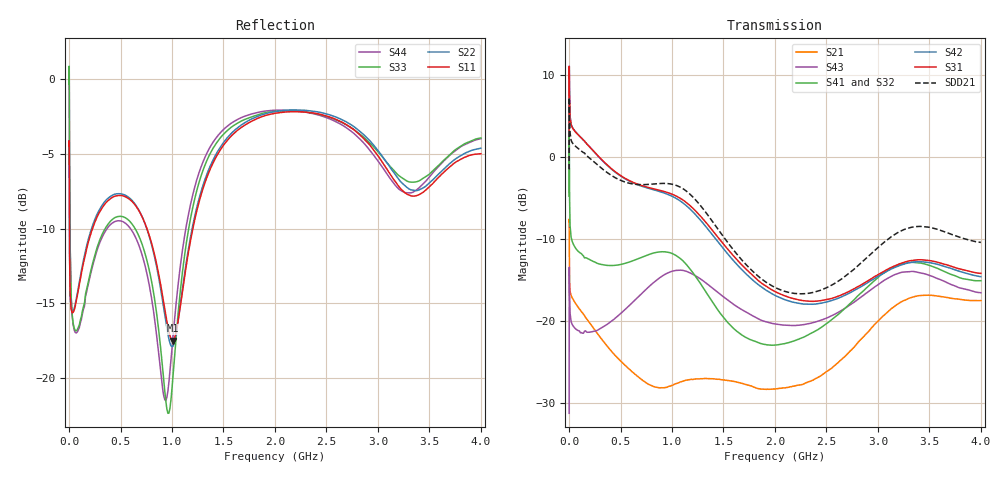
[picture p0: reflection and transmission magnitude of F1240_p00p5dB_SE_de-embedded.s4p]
! Integrated Device Technology
! Corporate Headquarters
! 6024 Silver Creek Valley Road
! San Jose, CA 95138  USA
! Phone:  1-408-284-8200
! Toll Free:  1-800-223-1366
! Webpage:  http://www.idt.com/
! Timing and RF Division
! 515 Groton Road, Suite 102
! Westford, MA 01886-6024
! Device:  F1240
! Description: Dual Intermediate Frequency Digital Variable Gain Amplifier
! Frequency:  10.0 -  500.00 MHz
! Package:  5x5 mm QFN Plastic Package: 32 pin
! Ports:  8 RF, 20 DC
!  Pin  1  = GA3 / Data  Pin 17  = RF OUT_B+
!  Pin  2  = GA4 / CLK  Pin 18  = RF OUT_B-
!  Pin  3  = GA5  Pin 19  = STBY_B
!  Pin  4  = VMODE  Pin 20  = Ground
!  Pin  5  = No Connect  Pin 21  = Ground
!  Pin  6  = GB5  Pin 22  = STB_A
!  Pin  7  = GB4  Pin 23  = RF OUT_A-  = Port 4
!  Pin  8  = GB3  Pin 24  = RF OUT_A+  = Port 3
!  Pin  9  = GB2  Pin 25  = GA0
!  Pin 10  = GB1  Pin 26  = ISET_A
!  Pin 11  = RF IN_B+  Pin 27  = VCC
!  Pin 12  = RF IN_B-  Pin 28  = Ground
!  Pin 13  = Ground  Pin 29  = RF IN_A-  = Port 2
!  Pin 14  = VCC  Pin 30  = RF IN_A+  = Port 1
!  Pin 15  = ISET_B  Pin 31  = GA1
!  Pin 16  = GB0  Pin 32  = GA2 / CSb
! Gain  = +19.5 dB
! State  = 1
! Voltage  = +5.00 V
! Current  = 85.292 mA (one channel only)
! Temperture  =  +25 C
! Test Date  =  2017-10-18
! Board  =  EB4031
! Data:  The device was measured on a custom evaluation board which has
!  individual transmission lines to the RF pins.  Data was collected
!  using a calibrated network analyzer.  The evaluation board was
!  de-embedded using Automatic Fixture Removal.
!  The reference plane is the edge of the package pin.
!  Only Channel A was measured.
!  This data is in single-ended operation.  If your needs are balanced
!  or differential S-parameters then this file needs to be used a
!  linear simulator.
! File Date:  2017-11-10  MJV
! Note:
!  Integrated Device Technology supplies this data as a sample of measured
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# Hz S dB R 100
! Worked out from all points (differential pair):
!   410 points, 500 kHz to 4 GHz, reference 100 ohm
!   strongest paths, dB at 500 kHz, 930 MHz, 1.96 GHz, 2.98 GHz, 4 GHz:
!     S31: 3.0, -4.2, -16.1, -14.5, -14.2
!     S42: 3.0, -4.4, -16.6, -14.7, -14.6
!     S41: -4.8, -11.6, -23.0, -14.9, -15.1
!     S32: -4.8, -11.8, -22.9, -15.3, -15.6
!     S43: -31.3, -14.3, -20.3, -15.8, -16.6
!     S21: -7.9, -28.2, -28.3, -20.3, -17.5
!   taken as a pair (ports 1,2 in; 3,4 out), SDD21 dB: -1.5, -3.2, -15.6, -11.3, -10.4
!   lowest |S11| = -17.5 dB at 1.01 GHz (marker M1), VSWR 1.31, Z = 78.1 - j9.33 ohm
!   |S11| at or under -10 dB: 3.776 MHz to 228.1 MHz (224.3 MHz wide, 193 % of centre); 756.2 MHz to 1.203 GHz (446.6 MHz wide, 45.6 % of centre)
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500000  -4.49 -5.6  -7.89 -5.8  -29.85 81.1  -37.54 79.1
        -7.89 -5.7  -4.48 -5.6  -37.51 78.1  -29.87 82.3
        3.04 -107.0  -4.75 -109.0  -0.33 0.9  -31.31 -47.4
        -4.77 -107.9  3.03 -105.9  -31.28 -47.5  -0.33 3.2
2500000  -7.21 -43.9  -11.72 -41.1  -19.66 24.5  -29.11 0.8
         -11.73 -41.1  -7.19 -44.0  -29.08 0.6  -19.66 24.7
         10.38 177.2  1.11 154.7  -1.00 -58.1  -13.59 -155.8
         1.07 154.9  10.37 177.4  -13.58 -155.8  -1.05 -57.8
4500000  -11.09 -46.1  -15.06 -31.1  -19.87 9.5  -31.70 -11.8
         -15.07 -31.1  -11.07 -46.4  -31.67 -11.9  -19.87 9.6
         7.62 161.4  -4.21 139.1  -5.19 -84.2  -16.19 174.0
         -4.26 139.2  7.62 161.5  -16.17 173.9  -5.24 -84.2
1.7e8  -11.37 -107.4  -19.72 -53.6  -22.05 -44.1  -35.47 -28.1
       -19.73 -53.5  -11.18 -108.7  -35.55 -27.7  -22.06 -44.4
       1.64 116.5  -12.35 80.8  -14.10 -142.6  -21.41 106.7
       -12.32 80.6  1.64 115.8  -21.36 106.2  -14.25 -142.4
5.3e8  -7.82 -164.0  -25.27 -114.5  -23.62 -109.3  -33.62 -76.6
       -25.25 -113.9  -7.72 -165.6  -33.80 -74.5  -23.82 -109.7
       -2.49 23.8  -13.13 -47.5  -9.22 -172.8  -18.95 6.9
       -13.02 -48.8  -2.55 22.5  -18.77 6.6  -9.56 -173.3
1.01e9  -17.51 -153.9  -28.18 -157.4  -22.61 148.6  -30.84 -167.5
        -27.84 -159.8  -17.88 -151.1  -30.82 -161.8  -23.25 147.5
        -4.58 -93.4  -12.02 165.3  -19.83 -115.0  -14.15 -119.6
        -11.82 161.4  -4.84 -95.9  -13.91 -119.8  -17.21 -107.6
4e9  -4.99 -141.1  -17.55 105.0  -23.96 -41.9  -24.95 -25.8
     -17.52 104.8  -4.62 -139.4  -25.85 -10.4  -25.70 -35.0
     -14.20 40.4  -15.57 -63.1  -3.93 -134.2  -18.01 66.5
     -15.09 -76.7  -14.60 46.3  -16.56 57.7  -3.98 -143.9
